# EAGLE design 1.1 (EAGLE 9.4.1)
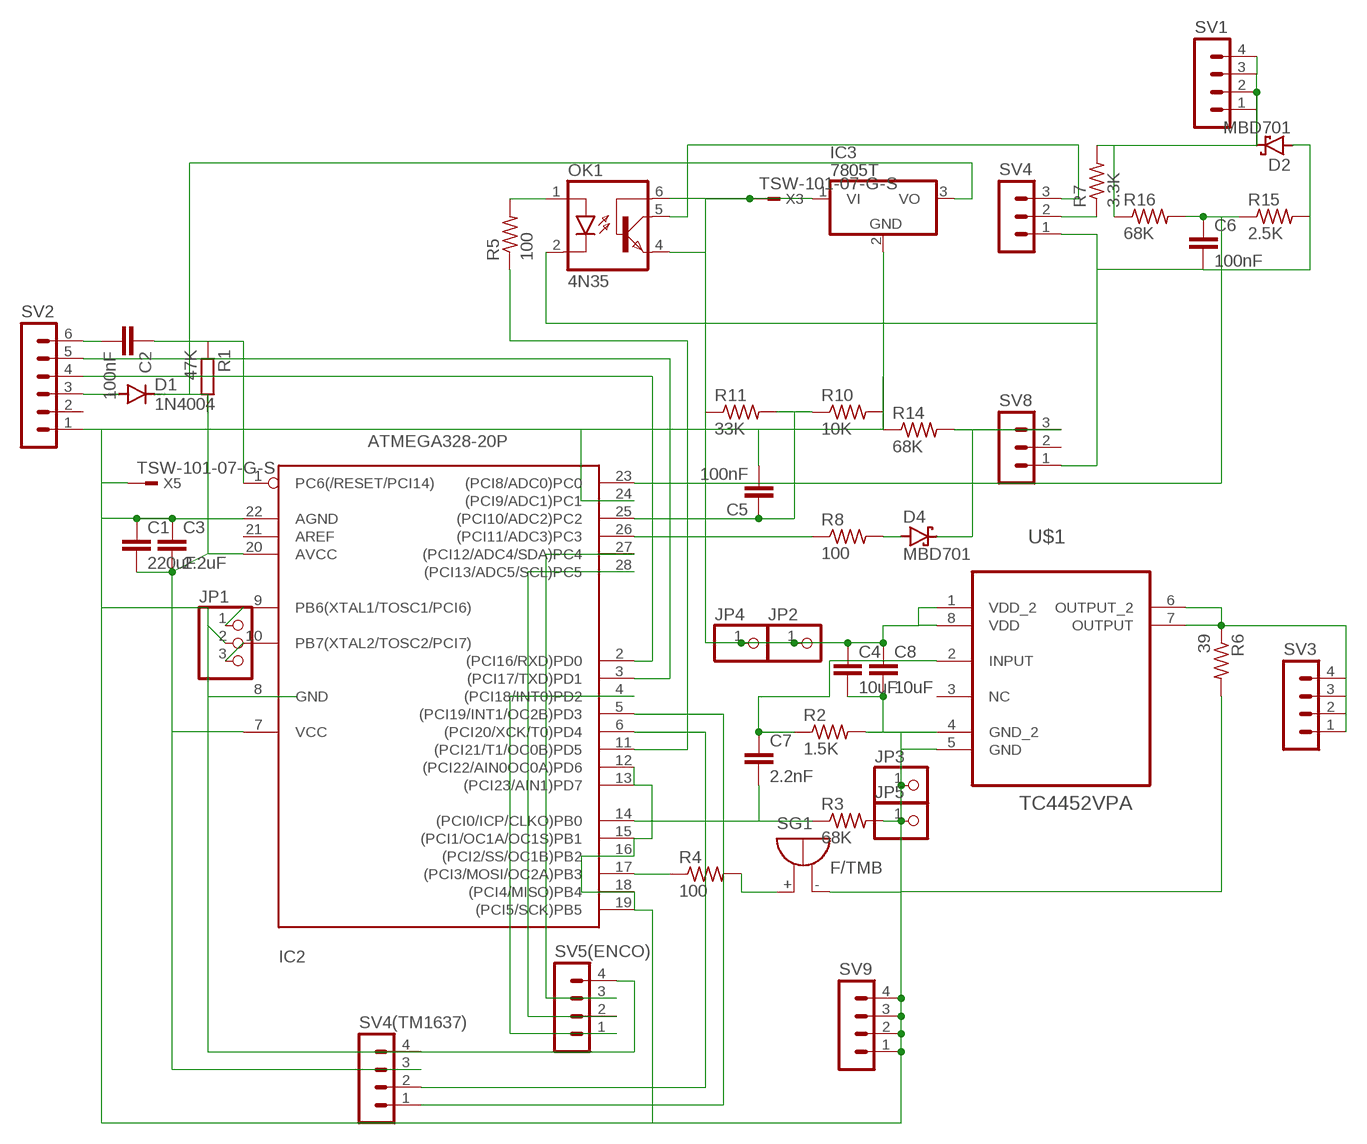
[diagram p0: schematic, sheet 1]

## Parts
C1  220uF  C2.5/2  [C2.5-2]
C2  100nF  C5/7.2  [C5B7.2]
C3  2.2uF  C2.5/2  [C2.5-2]
C4  10uF  C2.5/2  [C2.5-2]
C5  100nF  C2.5/4  [C2.5-4]
C6  100nF  C2.5/4  [C2.5-4]
C7  2.2nF  C2.5/4  [C2.5-4]
C8  10uF  C2.5/2  [C2.5-2]
D1  1N4004  [DO41-10]
D2  MBD701  [TO92H]
D4  MBD701  [TO92H]
IC2  ATMEGA328-20P  [DIL28-3]
IC3  7805T  [TO220H]
JP1  PINHD-1X3  [1X03]
JP2  PINHD-1X1  [1X01]
JP3  PINHD-1X1  [1X01]
JP4  PINHD-1X1  [1X01]
JP5  PINHD-1X1  [1X01]
OK1  4N35  [DIL06]
R1  47K  R-EU_0204/7  [0204/7]
R2  1.5K  R-US_0204/2V  [0204V]
R3  68K  R-US_0204/2V  [0204V]
R4  100  R-US_0204/2V  [0204V]
R5  100  R-US_0204/2V  [0204V]
R6  39  R-US_0204/2V  [0204V]
R7  3.3K  R-US_0204/2V  [0204V]
R8  100  R-US_0204/2V  [0204V]
R10  10K  R-US_0204/2V  [0204V]
R11  33K  R-US_0204/2V  [0204V]
R14  68K  R-US_0204/2V  [0204V]
R15  2.5K  R-US_0204/2V  [0204V]
R16  68K  R-US_0204/2V  [0204V]
SG1  F/TMB  [F/TMB]
SV1  MA04-1  [MA04-1]
SV2  MA06-1  [MA06-1]
SV3  MA04-1  [MA04-1]
SV4  MA03-1  [MA03-1]
SV4(TM1637)  MA04-1  [MA04-1]
SV5(ENCO)  MA04-1  [MA04-1]
SV8  MA03-1  [MA03-1]
SV9  MA04-1  [MA04-1]
U$1  TC4452VPA  [DIP254P762X432-8]
X3  TSW-101-07-G-S  [TSW-101-XX-G-S]
X5  TSW-101-07-G-S  [TSW-101-XX-G-S]

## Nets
N$2: IC2.11((PCI21/T1/OC0B)PD5) R5.1
N$3: IC2.17((PCI3/MOSI/OC2A)PB3) R4.1
N$4: R4.2 SG1.+
N$5: D1.A SV2.3
N$6: OK1.1(A) R5.2
N$7: IC2.2((PCI16/RXD)PD0) SV2.4
N$8: IC2.3((PCI17/TXD)PD1) SV2.5
N$9: C2.2 SV2.6
N$10: C2.1 IC2.1(PC6(/RESET/PCI14)) R1.1
N$11: C1.2 C3.2 D1.C IC2.7(VCC) IC2.20(AVCC) IC3.3(VO) R1.2 SV4(TM1637).3
N$12: C4.1 C8.1 IC3.1(VI) JP2.1 JP4.1 OK1.4(EMI) OK1.6(BAS) R11.1 U$1.1(VDD_2) U$1.8(VDD) X3.1
N$13: R6.1 SV3.1 SV3.2 SV3.3 SV3.4 U$1.6(OUTPUT_2) U$1.7(OUTPUT)
N$14: D2.2(C) R7.2 R16.1 SV1.1 SV1.2 SV1.3 SV1.4
N$15: C7.2 IC2.14((PCI0/ICP/CLKO)PB0) R3.1
N$16: IC2.26((PCI11/ADC3)PC3) R8.1
N$17: C5.1 IC2.25((PCI10/ADC2)PC2) R10.1 R11.2
N$18: D4.2(C) R14.2 SV8.3
N$19: C1.1 C3.1 C4.2 C5.2 C6.2 C8.2 D2.1(A) IC2.8(GND) IC2.12((PCI22/AIN0OC0A)PD6) IC2.13((PCI23/AIN1)PD7) IC2.15((PCI1/OC1A/OC1S)PB1) IC2.16((PCI2/SS/OC1B)PB2) IC2.18((PCI4/MISO)PB4) IC2.19((PCI5/SCK)PB5) IC2.22(AGND) IC2.24((PCI9/ADC1)PC1) IC3.2(GND) JP1.2 JP3.1 JP5.1 OK1.2(C) R2.2 R3.2 R6.2 R10.2 R14.1 R15.2 SG1.- SV2.1 SV4(TM1637).4 SV4.1 SV5(ENCO).4 SV8.1 SV9.1 SV9.2 SV9.3 SV9.4 U$1.4(GND_2) U$1.5(GND)
N$20: IC2.6((PCI20/XCK/T0)PD4) SV4(TM1637).2
N$21: IC2.5((PCI19/INT1/OC2B)PD3) SV4(TM1637).1
N$22: R7.1 SV4.2
N$23: D4.1(A) R8.2
N$24: IC2.4((PCI18/INT0)PD2) SV5(ENCO).1
N$25: IC2.28((PCI13/ADC5/SCL)PC5) SV5(ENCO).2
N$26: IC2.27((PCI12/ADC4/SDA)PC4) SV5(ENCO).3
N$27: IC2.9(PB6(XTAL1/TOSC1/PCI6)) JP1.1
N$28: IC2.10(PB7(XTAL2/TOSC2/PCI7)) JP1.3
N$29: C6.1 IC2.23((PCI8/ADC0)PC0) R15.1 R16.2
N$30: X5.1
N$31: OK1.5(COL) SV4.3
N$35: C7.1 R2.1 U$1.2(INPUT)
Unconnected: IC2.21(AREF) SV2.2 SV8.2 U$1.3(NC)

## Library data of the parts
C1-C8 = capacitor-wima:C: CAPACITOR
D1 = diode:1N4004: DIODE
D2 D4 = diode:MBD701: UHF DIODE
IC2 = atmega328:ATMEGA328*P: MICROCONTROLLER 32 kBytes FLASH 2 kBytes SRAM 1 kBytes EEPROM USART 8-channel 10 bit ADC
IC3 = linear:78*: Positive VOLTAGE REGULATOR Source: http://cache.national.com/ds/LM/LM78L05.pdf http://www.fairchildsemi.com/ds/LM/LM7805.pdf
JP1 = pinhead:PINHD-1X3: PIN HEADER
JP2-JP5 = pinhead:PINHD-1X1: PIN HEADER
OK1 = optocoupler:4N35: MOTOROLA OPTO COUPLER; MF: FAIRCHILD SEMICONDUCTOR; MPN: 4N35; OC_FARNELL: 1328375; OC_NEWARK: 72K9946
R1 = rcl:R-EU_: RESISTOR, European symbol; SPICEPREFIX: R
R2-R8 R10 R11 R14-R16 = rcl:R-US_: RESISTOR, American symbol; SPICEPREFIX: R
SG1 = buzzer:F/TMB: BUZZER; OC_FARNELL: unknown; OC_NEWARK: unknown
SV1 SV3 SV4(TM1637) SV5(ENCO) SV9 = con-lstb:MA04-1: PIN HEADER; OC_FARNELL: unknown; OC_NEWARK: unknown
SV2 = con-lstb:MA06-1: PIN HEADER; OC_FARNELL: unknown; OC_NEWARK: unknown
SV4 SV8 = con-lstb:MA03-1: PIN HEADER; OC_FARNELL: unknown; OC_NEWARK: unknown
U$1 = TC4452VPA:TC4452VPA: 12A High-Speed MOSFET Drivers; AVAILABILITY: Unavailable; DESCRIPTION: TC4452 Series 13 A 18 Vmax 1.5 Ohm Single Low Side MOSFET Driver - PDIP-8; MF: Microchip; MP: TC4452VPA; PACKAGE: PDIP-8 Microchip; PRICE: None
X3 X5 = con-samtec:TSW-101-*-G-S: THROUGH-HOLE .025" SQ POST HEADER; MF: Samtec Inc.; MPN: TSW-101-07-G-S

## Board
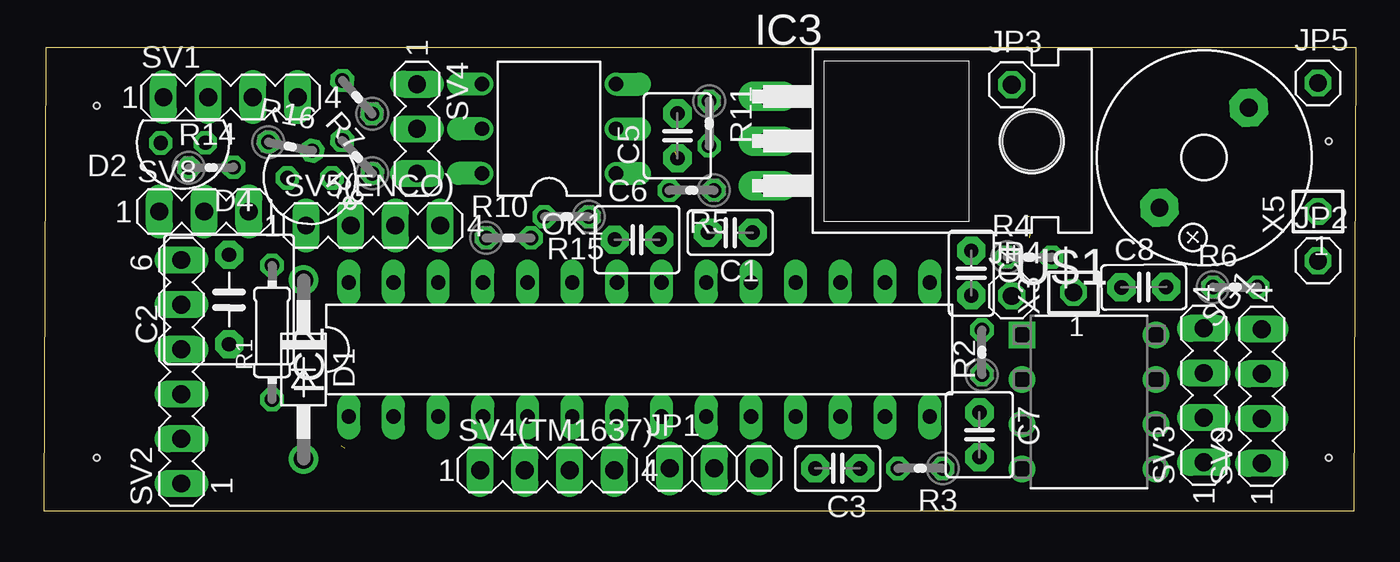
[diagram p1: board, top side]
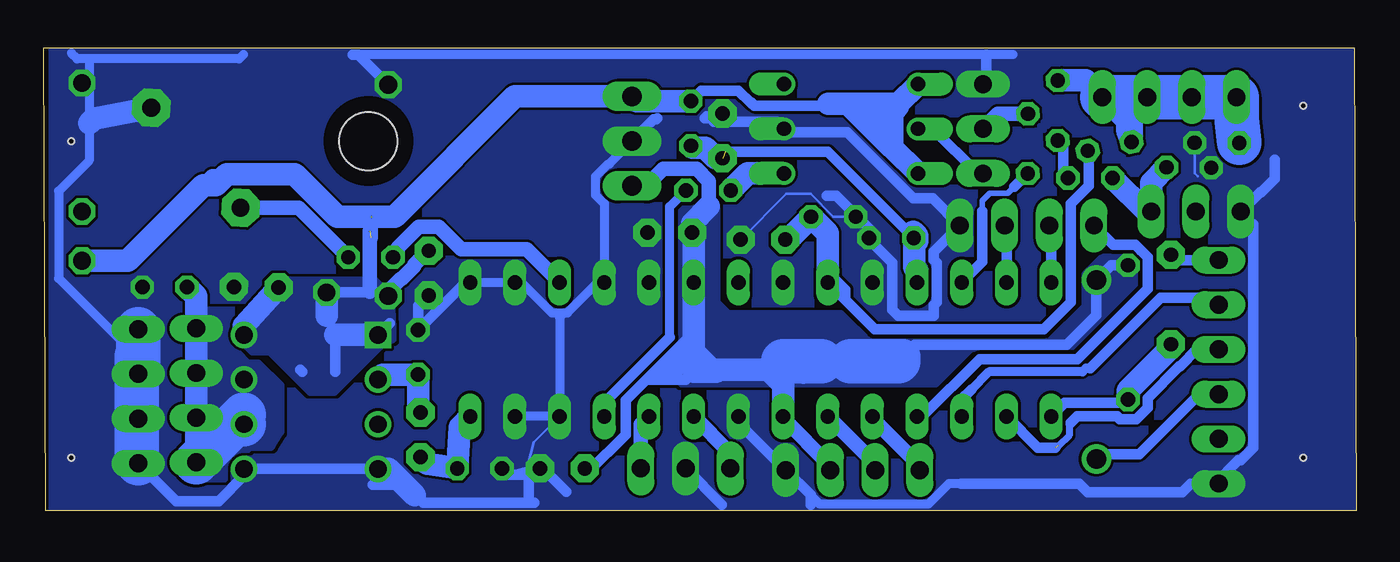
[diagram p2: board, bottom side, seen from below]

Size 74.56 x 26.3 mm. Coordinates in mm from the lower left corner, seen from the top.
Outline: 0,0 74.46,0 74.56,26.3 0.1,26.3 0,0
Copper layers (1*16): Top 0.035mm / dielectric 1.5mm / Bottom 0.035mm
Design rules "default *": minimum track width 6mil, minimum drill 0.35mm, track to track 6mil, track to pad 6mil, pad to pad 6mil, via to via 6mil, smd to smd 6mil, copper to edge 1mil, drill to drill 6mil, minimum pad ring 10mil, minimum via ring 8mil, stop-mask expansion 4mil, vias tented up to drill 0mil, thermal gap 10mil
Holes 0.35 mm at 3,3 3,23 73,3 73,21

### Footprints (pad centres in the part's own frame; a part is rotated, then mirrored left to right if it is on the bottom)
C2.5-2 = drill 0.813 pad 1.6 octagon: 1 -1.27,0; 2 1.27,0
C5B7.2 = drill 0.813 pad 1.6 octagon: 1 -2.54,0; 2 2.54,0
C2.5-4 = drill 0.813 pad 1.6 octagon: 1 -1.27,0; 2 1.27,0
DO41-10 = drill 1.118: A 5.08,0; C -5.08,0
TO92H = drill 0.813 octagon: 1 -1.27,0; 2 1.27,0
DIL28-3 = drill 0.813 long: 1 -16.51,-3.81; 2 -13.97,-3.81; 3 -11.43,-3.81; 4 -8.89,-3.81; 5 -6.35,-3.81; 6 -3.81,-3.81; 7 -1.27,-3.81; 8 1.27,-3.81; 9 3.81,-3.81; 10 6.35,-3.81; 11 8.89,-3.81; 12 11.43,-3.81; 13 13.97,-3.81; 14 16.51,-3.81; 15 16.51,3.81; 16 13.97,3.81; 17 11.43,3.81; 18 8.89,3.81; 19 6.35,3.81; 20 3.81,3.81; 21 1.27,3.81; 22 -1.27,3.81; 23 -3.81,3.81; 24 -6.35,3.81; 25 -8.89,3.81; 26 -11.43,3.81; 27 -13.97,3.81; 28 -16.51,3.81
TO220H = drill 1.118 long: 1 -2.54,-10.16; 2 0,-10.16; 3 2.54,-10.16 | hole 3.302: 0,4.826
1X03 = drill 1.016 long: 1 -2.54,0; 2 0,0; 3 2.54,0
1X01 = drill 1.016 octagon: 1 0,0
DIL06 = drill 0.813 offset: 1 -2.54,-3.81; 2 0,-3.81; 3 2.54,-3.81; 4 2.54,3.81; 5 0,3.81; 6 -2.54,3.81
0204/7 = drill 0.813 octagon: 1 -3.81,0; 2 3.81,0
0204V = drill 0.813 octagon: 1 -1.27,0; 2 1.27,0
F/TMB = drill 1.016 pad 2.159 octagon: + 3.81,0; - -3.81,0
MA04-1 = drill 1.016 long: 1 -3.81,0; 2 -1.27,0; 3 1.27,0; 4 3.81,0
MA06-1 = drill 1.016 long: 1 -6.35,0; 2 -3.81,0; 3 -1.27,0; 4 1.27,0; 5 3.81,0; 6 6.35,0
MA03-1 = drill 1.016 long: 1 -2.54,0; 2 0,0; 3 2.54,0
DIP254P762X432-8 = drill 0.991 square: 1 -7.62,7.62 | drill 0.991: 2 -7.62,5.08; 3 -7.62,2.54; 4 -7.62,0; 5 0,0; 6 0,2.54; 7 0,5.08; 8 0,7.62
TSW-101-XX-G-S = drill 1 pad 1.5 octagon: 1 0,0

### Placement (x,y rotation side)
C1  39,15.8 180 top
C2  10.52,12 90 top
C3  45.1,2.4 180 top
C4  52.7,13.5 270 top
C5  36,21.3 90 top
C6  33.7,15.4 0 top
C7  53.16,4.31 270 top
C8  62.5,12.7 0.7 top
D1  14.75,8.02 270 top
D2  7.9,20.9 180.1 top
D4  15.1,18.9 180 top
IC2  33.83,9.16 0 top
IC3  51.3,21 270 top
JP1  38.1,2.4 0 top
JP2  72.4,14.2 0 top
JP3  55,24.2 0 top
JP4  55,12.2 0 top
JP5  72.4,24.3 0 top
OK1  28.7,21.7 90 top
R1  12.96,10.13 90 top
R2  53.3,9 90 top
R3  49.8,2.4 180 top
R4  56,14.4 0 top
R5  36.8,18.2 180 top
R6  67.7,12.7 0 top
R7  17.8,23.5 131.8 top
R8  17.8,20.1 132.3 top
R10  26.4,15.5 0 top
R11  37.8,22 270 top
R14  9.5,19.5 0.7 top
R15  29.7,16.7 180 top
R16  14,20.7 348.8 top
SG1  65.93,20.06 228.2 top
SV1  10.6,23.5 0 top
SV2  7.81,7.89 90 top
SV3  65.91,6.55 90 top
SV4  21.2,21.7 270 top
SV4(TM1637)  28.6,2.3 0 top
SV5(ENCO)  18.7,16.2 0 top
SV8  9.1,17 0 top
SV9  69.2,6.5 90 top
U$1  63.2,2.37 0 top
X3  58.5,12.4 0 top
X5  72.4,17 0 top

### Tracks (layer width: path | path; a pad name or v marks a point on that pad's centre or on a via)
N$2
  Bottom 0.508: R5.1 39,17.27 39,9.85
  Bottom 0.61: 39,9.85 42.72,6.13 IC2.11
N$3
  Bottom 0.61: R4.1 54.73,14.22
  Bottom 0.813: R4.1 54.46,14.67 54.46,14.93 53.26,16.13 52.14,16.13 50.86,14.85 47.14,14.85 IC2.17
N$4
  Bottom 0.813: R4.2 60.09,17.22 SG1.+
N$5
  Bottom 0.61: SV2.3 8.91,6.62 12.32,3.21 14.48,3.21 D1.A
N$6
  Bottom 1.27: OK1.1 34.57,19.16 R5.2
N$7  (1 unrouted)
  Bottom 0.406: 16.2,5 16.3,4.9 16.3,4.27 16.9,3.67 | SV2.4 8.71,9.16
  Bottom 0.61: 19.56,5.35 IC2.2 18.08,3.57 17.1,3.57 | SV2.4 9.04,9.16 10,8.2 10.03,8.2 11.84,6.39 11.84,5.86 12.5,5.2 13.42,5.2 13.58,5.36 15.84,5.36 16.2,5
N$8
  Bottom 0.508: 15.11,8.11 15.33,8.11 15.55,7.89 20.86,7.89 21.88,6.88
  Bottom 0.61: IC2.3 22.4,6.35 21.88,6.88 | SV2.5 8.21,12.1 11.11,12.1 15.11,8.11
N$9
  Bottom 0.61: SV2.6 10.22,14.24 C2.2
N$10
  Bottom 0.61: IC2.1 16.55,6.12 13.16,6.12 R1.1
  Bottom 1.27: R1.1 12.96,6.82 10.52,9.26 C2.1
N$11
  Bottom 0.508: IC2.7 32.56,6.62 33.83,7.89 | 33.83,7.89 36.37,7.89 | 32.56,7.89 33.83,7.89
  Bottom 0.61: 30.4,8.5 31.4,7.5 | 37.64,13.2 IC2.20 37.64,13.34 | R1.2 13.91,13.94 D1.C 14.75,11.1 16.44,9.41 25.09,9.41 26,8.5 | C3.2 43.59,2.22 41.5,4.32 41.5,6.27 39.88,7.88 | 37.64,7.89 38.1,7.43 39,7.43 | 38.36,9.36 40.3,7.43 39,7.43 | 38.36,9.36 38,9.73 38,9.77 39.88,7.88 | 38.36,9 38.36,8.06 | 38.36,9 38.36,9.36 | 39.88,7.88 39.48,7.88 39.18,8.18 | 39.18,8.18 38.36,9 | 39,7.43 38.36,8.06 | 38.36,8.06 39.06,8.06 39.18,8.18
  Bottom 0.813: 36.77,17.3 36.77,18.72 37.47,19.42 39.38,19.42 40.33,18.46 IC3.3 | SV4(TM1637).3 29.87,2.56 32.56,5.25 IC2.7
  Bottom 1.27: 37.64,9 37.64,7.89 36.37,7.89 | 37.64,9 IC2.20 37.64,15.76 C1.2 37.73,16.34 36.77,17.3 | IC2.7 32.56,7.89 32.56,8.5 | 37.64,9 36.64,8 33,8
  Bottom 2: 25.75,8.75 26,8.5
  Bottom 2.54: 32.56,8.5 30.4,8.5 | 26,8.5 28.7,8.5
  pour Bottom (isolate 0.21, no thermals): 38.3,7.3 38.3,17.1 36.4,17.1 36.4,11.8 35.7,11.1 29.3,11.1 27.7,9.5 17.4,9.5 15.3,11.6 15.3,13.4 14.4,14.3 12.9,14.3 12.7,14.1 12.7,12.8 16.2,9.3 21.9,9.3 23.9,7.3
N$12  (2 unrouted)
  Bottom 0.152: 55.28,10.29 U$1.1 | OK1.6 25.16,19.16
  Bottom 0.61: 60,8 59.89,7.89 | 58,9.99 58,7.89 | OK1.6 26,20.27 | 26,20.27 26.1,20.37 26.1,22.9 | 26,20.27 26,20.17 28.95,23.12 30,23.12 30.1,23.02 34.19,23.02 34.29,23.12 34.35,23.12 34.41,23.18 | 26,23 24.89,24.11 OK1.4 | R11.1 37.2,23.87 35.1,23.87 34.41,23.18 | 34.35,23.18 34.41,23.18 | 54.91,10.66 55.28,10.29 | JP4.1 55.2,12.4 56,12.4 | 56,12.4 X3.1 | 56.05,12.45 56,12.4
  Bottom 0.813: 56.05,15.89 56.05,12.45 | 56,15.5 56,16.7 | 65.5,18.5 65,19 62.79,19 | JP4.1 55,12.47 54.29,13.18 54.23,13.18 53.51,13.89 53.51,13.96 C4.1
  Bottom 1.27: U$1.1 58,9.99 | U$1.8 63.2,10.52 C8.1 | OK1.6 26.36,20.64 | 26.36,20.64 27.36,21.64 | 27.36,21.64 28.85,23.12 | 28.85,23.12 30,23.12 | OK1.4 26.01,23.12 27,23.12 | 28.85,23.12 27,23.12 | 26,23 26.1,22.9 26.36,22.64 26.36,20.64 | 27.36,21.64 27,22 27,23.12 | R11.1 40.87,23.27 IC3.1 47.8,23.54 54.64,16.7 56,16.7 | 58.5,11.07 X3.1 | 55.9,16.7 57.88,16.7 60.31,19.13 64.17,19.13 64.8,18.5 65.5,18.5 69.8,14.2 JP2.1
  pour Bottom (no thermals): 54.79,9.8 55.1,9.8 58.1,6.8 59.4,6.8 61.7,9.1 62.7,9.1 62.9,9.3 62.9,11 60.9,13 55.8,13 54.9,12.1
N$13
  Bottom 1.27: SV3.1 SV3.2 SV3.3 SV3.4 65.91,12.18 R6.1
  Bottom 2.54: 63.21,5.44 SV3.1 63.74,4.91 U$1.6
  pour Bottom (no thermals): 61.2,4.5 61.2,7.1 62.4,8.3 63,8.3 63.7,9 63.7,11.2 63.8,11.3 66,11.3 66.1,11.2 66.1,2 66,1.9 63.8,1.9 63.4,2.3 63.4,3.2 62.9,3.7 61.7,3.7
N$14
  Bottom 0.508: SV1.3 SV1.2 9.83,23 | SV1.4 13.81,22.9 10.63,22.9
  Bottom 0.61: SV1.2 SV1.1 | SV1.4 13.95,23.04 | R16.1 12.66,21.33 16.11,24.77 R7.2
  Bottom 1.27: R7.2 15.36,24.45 SV1.4 | 13,23.5 13,21.61 R16.1 12.74,22.62 SV1.3
  Bottom 2.54: SV1.4 13,23.5 SV1.3 SV1.1 6.79,22.19 D2.2
N$15
  Bottom 0.61: R3.1 50.84,4.74
  Bottom 1.27: C7.2 52.78,2.66 R3.1 50.94,4.75 IC2.14
N$16
  Bottom 0.305: 19.41,18.41 19.79,18.03 20.81,18.03 21.24,17.6 21.24,17
  Bottom 0.61: IC2.26 21.24,14.13 21.24,17 | R8.1 19.41,18.41
N$17  (1 unrouted)
  Bottom 0.152: 25.16,15.84 25.16,15.54 R10.1
  Bottom 0.61: R10.1 30.01,20.38 35.85,20.38 | R11.2 37.6,20.93
  Bottom 1.27: R11.2 37.68,20.61 36.97,20.61 36.39,20.03 C5.1 | 25.16,15.84 24.94,15.61 24.94,15.31 25.09,15.16 25.09,13.82 24.94,13.67 IC2.25
N$18
  Bottom 1.27: R14.2 11.64,18.64 SV8.3 11.93,17 D4.2
N$19
  Bottom 0.152: R15.2 29.7,16.7 31,18 32.37,18 C6.2 | D2.1 9.17,19.17 9,19 | IC2.12 46.72,3.89 47.2,2.05 | R3.2 48.6,2.05 | 47.2,2.05 | 35.26,22.59 35.81,22.59
  Bottom 0.508: 73,26 72.67,25.67 72,25.67 | 72,25.67 63.47,25.67 63.23,25.91 | 19.5,25.91 21,25.91 57,25.91 | 72,25.67 72,22 72,19.89 73.73,18.16 73.73,13.2 69.3,8.77 68.75,8.22 | IC3.2 42.44,19.7 42.49,19.7 43.22,18.98 43.22,17.94 42.72,17.44 IC2.18 43.09,12.97 44.82,11.24 45,11.24 | IC2.15 IC2.16 47.43,12.97 45.7,11.24 45,11.24 | 45,11.24 45.26,10.98 IC2.12 IC2.13 | 21,1.54 23.14,1.54 24.31,0.37 30.48,0.37 SV4(TM1637).4
  Bottom 0.61: 36.3,22.3 36.5,22.1 32.91,22.1 OK1.2 | 36.3,22.3 36.18,22.42 36.88,22.42 37,22.3 36.3,22.3 | 4.62,19.94 4.62,18.86 5.38,18.11 5.46,18.11 SV8.1 | 46.69,0.46 47,0.46 | 47,0.46 53,0.46 54,1.46 | 54,1.46 55.88,1.46 | SV9.3 69.2,6.73 | SV9.2 69.04,5.23 SV9.1 67.05,0.54 64.64,0.54 63.2,1.97 U$1.5 U$1.4 | SV9.4 68.56,10.96 | 40.18,13.49 IC2.19 | SV2.1 8,1.54 | 8,1.54 9.39,1.54 9.88,1.05 15.24,1.05 15.73,1.54 21,1.54 22.43,1.54 | 54.1,1.56 54,1.46 | IC2.22 | 39.71,22.3 39.77,22.25 39.9,22.25 IC3.2 | 32.31,21.5 28.91,21.5 25.15,17.74 24.05,17.74 SV5(ENCO).4 24,14.71 24,14.27 23.82,14.09 23.82,11.85 24,11.67 24,11.06 26,11.06 26.36,11.42 26.36,14.09 27.67,15.4 R10.2 27.67,16.01 29.54,17.88 30.08,17.88 | 5.83,14.75 5.83,14.74 | 5.83,14.74 5.83,3.58 6.54,2.86 6.68,2.86 8,1.54 | 21,24.44 21,25.91 | 5.83,16.27 5.83,14.74 | JP1.2 36.03,0.33 | 31,0.33 31,0.89 SV4(TM1637).4 35.1,4.99 IC2.8 | 44.87,1.07 46.3,2.51 C3.1 47.7,2.05 | IC2.15 50.6,12.97 R2.2 53.3,11.63 C4.2 | 47,0.46 47,1.85 47.2,2.05 47.7,2.05 | 47.7,2.05 48.6,2.05 | JP3.1 56.71,25.91 57,25.91
  Bottom 1.27: U$1.4 55,2.37 53.5,0.87 | SG1.- 71.73,22.27 72,22
  Bottom 2.54: SV9.4 SV9.3 SV9.4 | 69.3,8.77 69.3,2.79 SV9.1
  pour Bottom (rank 6, no thermals): 0,26.2 74,26.2 74,0 0,0
N$20
  Bottom 0.813: SV4(TM1637).2 27.33,2.66 IC2.6
N$21
  Bottom 0.813: SV4(TM1637).1 24.79,2.56 27.48,5.25 IC2.5
N$22
  Bottom 0.813: R7.1 20.35,22.55 SV4.2
N$23
  Bottom 0.61: D4.1 16.64,19.18 16.64,20.74 R8.2
N$24
  Bottom 0.406: 12.29,14.71 11.94,14.36 11.94,12.5
  Bottom 0.61: IC2.4 24.64,5.35 21.39,8.6 15.84,8.6 11.94,12.5 11.84,12.6 11.84,14.4 12.54,15.1 13.79,15.1 SV5(ENCO).1
N$25
  Bottom 0.152: 17.32,16.09 SV5(ENCO).2
  Bottom 0.61: IC2.28 17.32,16.09
N$26
  Bottom 0.152: 19.89,16.11 SV5(ENCO).3
  Bottom 0.61: IC2.27 19.86,16.09 19.89,16.11
N$27
  Bottom 0.813: JP1.1 35.56,3.27 IC2.9
N$28
  Bottom 0.813: JP1.3 40.64,3.95 40.63,3.96 40.63,4.9 IC2.10
N$29
  Bottom 0.152: IC2.23 30.02,13
  Bottom 0.61: 32.36,15.31 32.45,15.4 C6.1 32.43,15.74 | 29.02,11.97 IC2.23 29.73,13.26 29.02,12.55 29.02,11.97 | 29.02,11.97 27.35,10.3 17.75,10.3 16.2,11.85 16.2,15.03 16.21,15.03 16.21,17.44 15.19,18.46 15.19,20.37 R16.2
  Bottom 1.27: 32.36,15.31 R15.1 30.02,15.75 IC2.23
N$31
  Bottom 0.61: 23.69,21.7 OK1.5 24.04,21.7 21.5,19.16 SV4.3
N$35
  Bottom 1.27: U$1.2 55.3,7.73 R2.1 53.3,5.5 C7.1
(copper drawn outside any net)
  shapes: Bottom area x1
